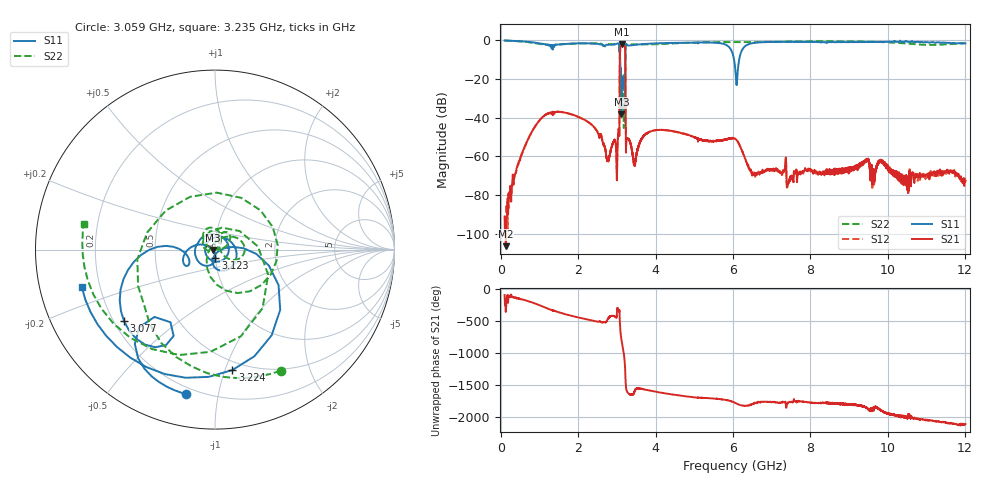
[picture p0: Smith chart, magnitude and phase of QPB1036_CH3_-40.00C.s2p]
! TDS: K:\Engsetup\Winsaw\QPB1036_ALL
! Channel 1
! Ports=1 2
! seg 1=100.000000 1100.000000 101
! seg 2=1101.000000 1501.000000 401
! seg 3=1502.000000 2502.000000 101
! seg 4=2503.000000 3803.000000 1301
! seg 5=3804.000000 5004.000000 121
! seg 6=5005.000000 6005.000000 1001
! seg 7=6006.000000 8406.000000 241
! seg 8=8407.000000 10607.000000 2201
! seg 9=10608.000000 12008.000000 141
! Points=5609
! FailCode=0
! Topology=ALL_SE(12)
!VNA Cal loaded =QPB1036_ALL_-40C
!PS1(V)= 5.000
!PS(mA)= 0.500
!PS2(V)= 0.630
!PS(mA)= -0.100
!PS3(V)= 1.170
!PS(mA)= 0.100
!PS4(V)= 1.170
!PS(mA)= -0.100
!Temp (C)= -40.00
# MHz S DB R 50
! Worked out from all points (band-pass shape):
!   5609 points, 100 MHz to 12.01 GHz, reference 50 ohm
!   highest |S21| = -2.16 dB at 3.132 GHz (marker M1); lowest = -106.2 dB at 130 MHz (marker M2)
!   |S21| within 3 dB of the highest: 3.085 GHz to 3.217 GHz (131.3 MHz wide, 4.17 % of centre)
!   lowest |S11| = -38.3 dB at 3.118 GHz (marker M3), VSWR 1.02, Z = 48.8 - j0.251 ohm
!   |S11| at or under -10 dB: 3.086 GHz to 3.219 GHz (132.9 MHz wide, 4.22 % of centre); 6.028 GHz to 6.163 GHz (134.7 MHz wide, 2.21 % of centre)
!   |S22| runs from -45.4 to -0.3 dB; largest |S21 - S12| = 0.0061
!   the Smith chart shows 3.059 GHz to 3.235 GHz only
!   S11 on the Smith chart (normalised r, x): 3.059 GHz: 0.16, -0.81; 3.077 GHz: 0.24, -0.33; 3.123 GHz: 1.00, -0.09; 3.224 GHz: 0.43, -1.06; 3.235 GHz: 0.13, -0.14
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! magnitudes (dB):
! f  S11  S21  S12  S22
! 100 MHz  -0.2  -90.9  -92.9  -0.3
! 130 MHz  -0.3  -106.2  -98.2  -0.3
! 1.127 GHz  -2.2  -38.9  -38.9  -2.3
! 2.092 GHz  -1.7  -40.4  -40.4  -1.8
! 2.769 GHz  -2.5  -61.2  -61.4  -2.1
! 3.002 GHz  -1.9  -72.3  -71.4  -1.8
! 3.059 GHz  -1.7  -48.0  -47.9  -2.3
! 3.077 GHz  -3.8  -11.5  -11.5  -9.8
! 3.118 GHz  -38.3  -2.3  -2.3  -22.8
! 3.123 GHz  -26.6  -2.2  -2.2  -28.3
! 3.132 GHz  -19.7  -2.2  -2.2  -28.1
! 3.195 GHz  -21.5  -3.0  -3.0  -18.1
! 3.224 GHz  -3.4  -19.7  -19.7  -4.2
! 3.235 GHz  -2.3  -57.4  -57.3  -2.5
! 3.259 GHz  -2.6  -50.8  -50.5  -2.3
! 3.454 GHz  -2.5  -63.7  -63.4  -2.3
! 4.074 GHz  -1.7  -46.4  -46.3  -2.2
! 6.056 GHz  -14.0  -51.0  -51.0  -1.1
! 6.626 GHz  -1.3  -68.3  -69.2  -1.0
! 8.046 GHz  -1.0  -67.5  -67.3  -0.6
! 10.02 GHz  -0.7  -67.0  -66.6  -1.2
! 12.01 GHz  -1.8  -72.6  -73.4  -1.6
